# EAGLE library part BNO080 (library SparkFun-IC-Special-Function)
Hillcrest Labs BNO080 - High Precision IMU (VR) The VR IMU uses the impressive BNO080 IMU. This IC has a combination triple axis accelerometer/gyro/magnetometer packaged with an ARM Cortex M0+ running powerful algorithms. The BNO080 Inertial Measurement Unit (IMU) produces accurate rotation vector headings, excellently suited for VR and other heading applications with a static rotation error of 2 degrees or less. It’s what we’ve been waiting for: all the sensor data is combined and drift corrected into meaningful, accurate IMU information. SparkFun Products: VR IMU (BNO080)
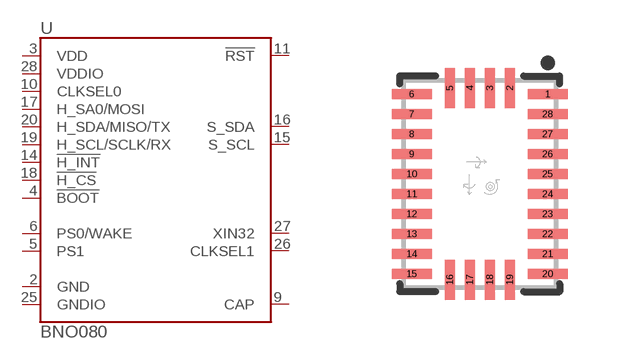
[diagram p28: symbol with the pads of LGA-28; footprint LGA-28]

Designator prefix U

## BNO080 (PROD_ID: SEN-13947)  [LGA-28]
2  GND
3  VDD
4  !BOOT
5  PS1
6  PS0/WAKE
9  CAP
10  CLKSEL0
11  !RST
14  !H_INT
15  S_SCL
16  S_SDA
17  H_SA0/MOSI
18  !H_CS
19  H_SCL/SCLK/RX
20  H_SDA/MISO/TX
25  GNDIO
26  CLKSEL1
27  XIN32
28  VDDIO

## Footprint LGA-28 (pad centres in mm)
LGA-28 - LGA-28 package for the BNO080 IMU Specifications: Pin count: 28 Pin pitch: 0.5mm Area: 3.8mm X 5.2mm Datasheet referenced for footprint Example device(s): BNO080
smd 1 x 0.25: 1 1.7,2.25; 6 -1.7,2.25; 7 -1.7,1.75; 8 -1.7,1.25; 9 -1.7,0.75; 10 -1.7,0.25; 11 -1.7,-0.25; 12 -1.7,-0.75; 13 -1.7,-1.25; 14 -1.7,-1.75; 15 -1.7,-2.25; 20 1.7,-2.25; 21 1.7,-1.75; 22 1.7,-1.25; 23 1.7,-0.75; 24 1.7,-0.25; 25 1.7,0.25; 26 1.7,0.75; 27 1.7,1.25; 28 1.7,1.75
smd 0.25 x 1: 2 0.75,2.4; 3 0.25,2.4; 4 -0.25,2.4; 5 -0.75,2.4; 16 -0.75,-2.4; 17 -0.25,-2.4; 18 0.25,-2.4; 19 0.75,-2.4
